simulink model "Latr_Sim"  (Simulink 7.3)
settings: Solver=ode45  StartTime=0.0  StopTime=40  MaxStep=0.01  RelTol=1e-4
InitFcn:
  | % Frequency Response Analysis file Run.m
  | d2r= pi/180; r2d=1/d2r;
  | LQR_des;
  | Mass=8878; Thr=320000;                          % Alpha Estimator parameters
  | Sref= 47.3; Qbar= 220; Cza=-0.31; Cyb=-0.06;
  | [Avf, Bvf, Cvf, Dvf]= vehi_latr_Sflx;          % Load Flex Vehicle Pitch Model
  | load -ascii KMIX.MAT KMIX;                          % Mixing Logic Matrix
  | load -ascii Klat.MAT Klat;                              % LQR Lateral State-Feedback Matrix
StopFcn:
  | Pl
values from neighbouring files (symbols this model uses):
  Aac = [    [actuator.m]
  Bac = [    [actuator.m]
  Cac = [    [actuator.m]
  Dac = [    [actuator.m]
undefined symbols (not defined in the file or in its folder): Avf, Bvf, Cvf, Dvf, Klat, KMIX

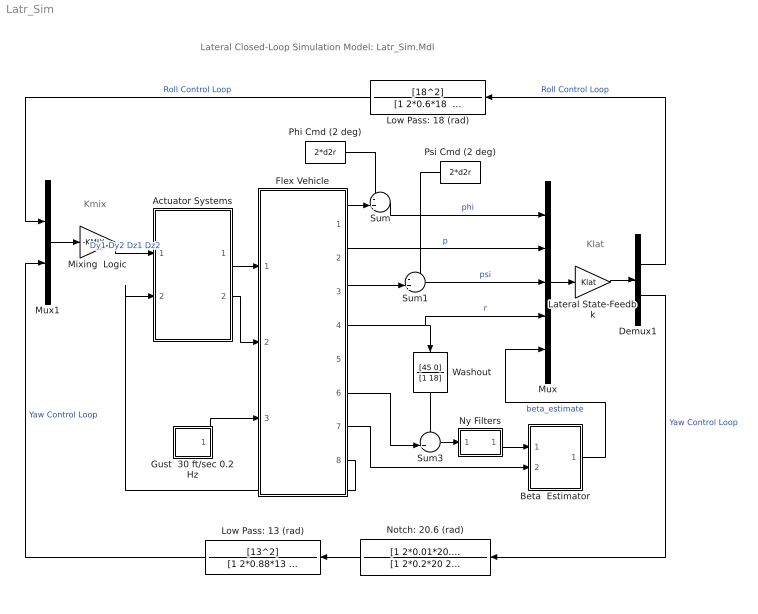
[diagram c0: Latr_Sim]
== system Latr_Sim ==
  note: Lateral Closed-Loop Simulation Model: Latr_Sim.Mdl
  note: Kmix
  note: Klat
  Actuator Systems : Subsystem
  Beta  Estimator : Subsystem
  Demux1 : Demux  Outputs=2
  Flex Vehicle : Subsystem
  Gust  30 ft/sec 0.2 Hz : Subsystem
  Lateral State-Feedbk : Gain  Gain=Klat  Multiplication=Matrix(K*u)  ParameterDataType=sfix(16)  ParameterScaling=2^0  OutDataType=sfix(16)  OutScaling=2^0
  Low Pass: 13 (rad) : TransferFcn  Numerator=[13^2]  Denominator="[1 2*0.88*13  13^2]"
  Low Pass: 18 (rad) : TransferFcn  Numerator=[18^2]  Denominator="[1 2*0.6*18  18^2]"
  Mixing  Logic : Gain  Gain=-KMIX  Multiplication=Matrix(K*u)  ParameterDataType=sfix(16)  ParameterScaling=2^0  OutDataType=sfix(16)  OutScaling=2^0
  Mux : Mux  Inputs=5
  Mux1 : Mux  Inputs=2
  Notch: 20.6 (rad) : TransferFcn  Numerator=[1 2*0.01*20.6 20.6^2]  Denominator=[1 2*0.2*20 20^2]
  Ny Filters : Subsystem
  Phi Cmd (2 deg) : Constant  Value=2*d2r  OutDataType=sfix(16)  OutScaling=2^0
  Psi Cmd (2 deg) : Constant  Value=2*d2r  OutDataType=sfix(16)  OutScaling=2^0
  Sum : Sum  Inputs=-+|  OutDataType=sfix(16)  OutScaling=2^0
  Sum1 : Sum  Inputs=-+|  OutDataType=sfix(16)  OutScaling=2^0
  Sum3 : Sum  Inputs=-+|  OutDataType=sfix(16)  OutScaling=2^0
  Washout : TransferFcn  Numerator=[45 0]  Denominator=[1 18]
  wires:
  Mux/1 -> Lateral State-Feedbk/1
  Lateral State-Feedbk/1 -> Demux1/1
  Mux1/1 -> Mixing  Logic/1
  Flex Vehicle/2(p) -> Mux/2  "p"
  Flex Vehicle/4(r) -> Mux/4, Washout/1  "r"
  Demux1/1 -> Low Pass: 18 (rad)/1  "Roll Control Loop"
  Low Pass: 18 (rad)/1 -> Mux1/1  "Roll Control Loop"
  Low Pass: 13 (rad)/1 -> Mux1/2  "Yaw Control Loop"
  Demux1/2 -> Notch: 20.6 (rad)/1  "Yaw Control Loop"
  Flex Vehicle/1(phi) -> Sum/2
  Sum/1 -> Mux/1  "phi"
  Flex Vehicle/3(psi) -> Sum1/2
  Sum1/1 -> Mux/3  "psi"
  Flex Vehicle/7(DZ) -> Beta  Estimator/2(Dz)
  Sum3/1 -> Ny Filters/1(In)
  Flex Vehicle/6(Ydd) -> Sum3/2
  Gust  30 ft/sec 0.2 Hz/1(Vgust) -> Flex Vehicle/3(Gust)
  Notch: 20.6 (rad)/1 -> Low Pass: 13 (rad)/1
  Ny Filters/1(out) -> Beta  Estimator/1(Ydd)
  Washout/1 -> Sum3/1
  Phi Cmd (2 deg)/1 -> Sum/1
  Psi Cmd (2 deg)/1 -> Sum1/1
  Beta  Estimator/1(bethat) -> Mux/5  "beta_estimate"
  Mixing  Logic/1 -> Actuator Systems/1(deltc)  "Dy1 Dy2 Dz1 Dz2"
  Actuator Systems/1(delta) -> Flex Vehicle/1(deltas)
  Actuator Systems/2(del_dd) -> Flex Vehicle/2(del_ddot)
  Flex Vehicle/8(TL) -> Actuator Systems/2(TL)

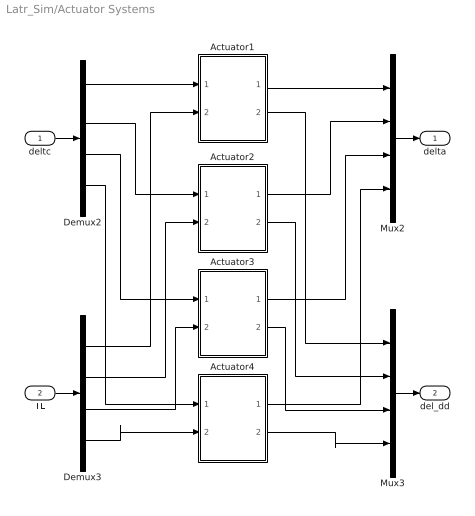
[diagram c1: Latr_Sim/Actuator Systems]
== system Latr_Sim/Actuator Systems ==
  deltc : Inport
  TL : Inport  Port=2
  Actuator1 : Subsystem
  Actuator2 : Subsystem
  Actuator3 : Subsystem
  Actuator4 : Subsystem
  Demux2 : Demux
  Demux3 : Demux
  Mux2 : Mux
  Mux3 : Mux
  delta : Outport
  del_dd : Outport  Port=2
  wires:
  Demux2/1 -> Actuator1/1(Dyc1)
  Demux2/2 -> Actuator2/1(Dyc2)
  Demux2/3 -> Actuator3/1(Dzc1)
  Demux2/4 -> Actuator4/1(Dzc2)
  Demux3/4 -> Actuator4/2(TLz2)
  Demux3/3 -> Actuator3/2(TLz1)
  Demux3/2 -> Actuator2/2(TLy2)
  Demux3/1 -> Actuator1/2(TLy1)
  Actuator1/1(Dy1) -> Mux2/1
  Actuator2/1(Dy2) -> Mux2/2
  Actuator3/1(Dz1) -> Mux2/3
  Actuator4/1(Dz2) -> Mux2/4
  Actuator4/2(Dz_dd2) -> Mux3/4
  Actuator3/2(Dz_dd1) -> Mux3/3
  Actuator2/2(Dy_dd2) -> Mux3/2
  Actuator1/2(Dy_dd1) -> Mux3/1
  deltc/1 -> Demux2/1
  Mux2/1 -> delta/1
  TL/1 -> Demux3/1
  Mux3/1 -> del_dd/1

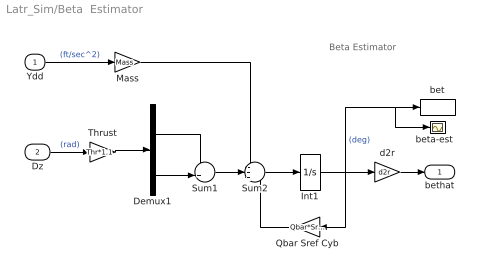
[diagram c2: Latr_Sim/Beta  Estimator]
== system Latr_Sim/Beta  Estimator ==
  note: Beta Estimator
  Ydd : Inport  OutDataType=sfix(16)  OutScaling=2^0
  Dz : Inport  Port=2  OutDataType=sfix(16)  OutScaling=2^0
  Demux1 : Demux  Outputs=2
  Int1 : Integrator
  Mass : Gain  Gain=Mass  ParameterDataType=sfix(16)  ParameterScaling=2^0  OutDataType=sfix(16)  OutScaling=2^0
  Qbar Sref Cyb : Gain  Gain=Qbar*Sref*Cyb  ParameterDataType=sfix(16)  ParameterScaling=2^0  OutDataType=sfix(16)  OutScaling=2^0
  Sum1 : Sum  Inputs=++|  OutDataType=sfix(16)  OutScaling=2^0
  Sum2 : Sum  Inputs=-++  OutDataType=sfix(16)  OutScaling=2^0
  Thrust : Gain  Gain=Thr*1.1  ParameterDataType=sfix(16)  ParameterScaling=2^0  OutDataType=sfix(16)  OutScaling=2^0
  bet : ToWorkspace  VariableName=bethat  SampleTime=-1  SaveFormat=Array
  "beta-est  " : Scope
  d2r : Gain  Gain=d2r  ParameterDataType=sfix(16)  ParameterScaling=2^0  OutDataType=sfix(16)  OutScaling=2^0
  bethat : Outport  OutDataType=sfix(16)  OutScaling=2^0
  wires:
  d2r/1 -> bethat/1
  Mass/1 -> Sum2/1
  Ydd/1 -> Mass/1  "(ft/sec^2)"
  Dz/1 -> Thrust/1  "(rad)"
  Qbar Sref Cyb/1 -> Sum2/3
  Int1/1 -> d2r/1, Qbar Sref Cyb/1, bet/1, "beta-est  "/1  "(deg)"
  Sum1/1 -> Sum2/2
  Sum2/1 -> Int1/1
  Thrust/1 -> Demux1/1
  Demux1/1 -> Sum1/1
  Demux1/2 -> Sum1/2

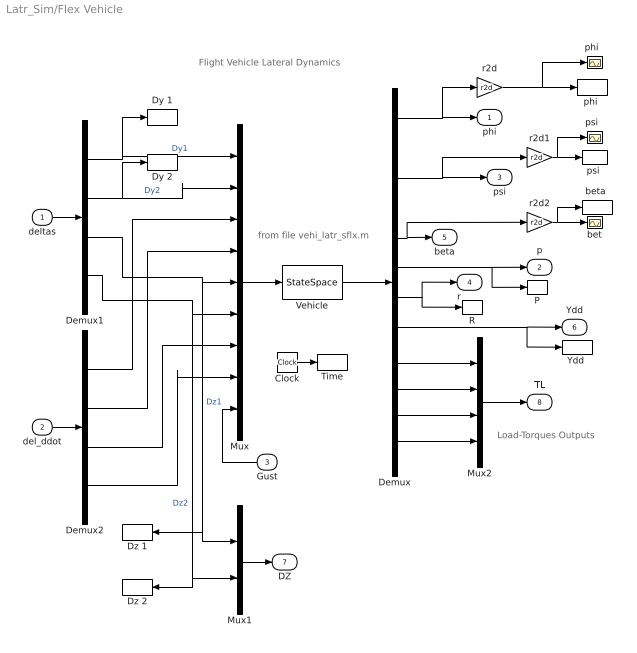
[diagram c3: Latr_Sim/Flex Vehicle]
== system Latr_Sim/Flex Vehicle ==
  note: Flight Vehicle Lateral Dynamics
  note: Load-Torques Outputs
  note: from file vehi_latr_sflx.m
  deltas : Inport  OutDataType=sfix(16)  OutScaling=2^0
  del_ddot : Inport  Port=2  OutDataType=sfix(16)  OutScaling=2^0
  Gust : Inport  Port=3  OutDataType=sfix(16)  OutScaling=2^0
  Clock : Clock
  Demux : Demux  Outputs=12
  Demux1 : Demux
  Demux2 : Demux
  Dy 1 : ToWorkspace  VariableName=Dy1  SampleTime=-1  SaveFormat=Array
  Dy 2 : ToWorkspace  VariableName=Dy2  SampleTime=-1  SaveFormat=Array
  Dz 1 : ToWorkspace  VariableName=Dz1  SampleTime=-1  SaveFormat=Array
  Dz 2 : ToWorkspace  VariableName=Dz2  SampleTime=-1  SaveFormat=Array
  Mux : Mux  Inputs=9
  Mux1 : Mux  Inputs=2
  Mux2 : Mux
  P : ToWorkspace  VariableName=p  SampleTime=-1  SaveFormat=Array
  R : ToWorkspace  VariableName=r  SampleTime=-1  SaveFormat=Array
  Time : ToWorkspace  VariableName=time  SampleTime=-1  SaveFormat=Array
  Vehicle : StateSpace  A=Avf  B=Bvf  C=Cvf  D=Dvf
  "Ydd " : ToWorkspace  VariableName=Ydd  SampleTime=-1  SaveFormat=Array
  bet : Scope
  "beta " : ToWorkspace  VariableName=beta  SampleTime=-1  SaveFormat=Array
  "phi " : ToWorkspace  VariableName=phi  SampleTime=-1  SaveFormat=Array
  "phi  " : Scope
  "psi " : ToWorkspace  VariableName=psi  SampleTime=-1  SaveFormat=Array
  "psi  " : Scope
  r2d : Gain  Gain=r2d  ParameterDataType=sfix(16)  ParameterScaling=2^0  OutDataType=sfix(16)  OutScaling=2^0
  r2d1 : Gain  Gain=r2d  ParameterDataType=sfix(16)  ParameterScaling=2^0  OutDataType=sfix(16)  OutScaling=2^0
  r2d2 : Gain  Gain=r2d  ParameterDataType=sfix(16)  ParameterScaling=2^0  OutDataType=sfix(16)  OutScaling=2^0
  phi : Outport  OutDataType=sfix(16)  OutScaling=2^0
  p : Outport  Port=2  OutDataType=sfix(16)  OutScaling=2^0
  psi : Outport  Port=3  OutDataType=sfix(16)  OutScaling=2^0
  r : Outport  Port=4  OutDataType=sfix(16)  OutScaling=2^0
  beta : Outport  Port=5  OutDataType=sfix(16)  OutScaling=2^0
  Ydd : Outport  Port=6  OutDataType=sfix(16)  OutScaling=2^0
  DZ : Outport  Port=7  OutDataType=sfix(16)  OutScaling=2^0
  TL : Outport  Port=8  OutDataType=sfix(16)  OutScaling=2^0
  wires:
  Mux/1 -> Vehicle/1
  Vehicle/1 -> Demux/1
  deltas/1 -> Demux1/1
  Demux1/1 -> Mux/1, Dy 1/1  "Dy1"
  Demux1/3 -> Mux/5, Mux1/1, Dz 1/1  "Dz1"
  Demux/1 -> phi/1, r2d/1
  Demux/3 -> psi/1, r2d1/1
  Demux/5 -> beta/1, r2d2/1
  Demux/8 -> Ydd/1, "Ydd "/1
  Demux/6 -> p/1, P/1
  Demux1/2 -> Mux/2, Dy 2/1  "Dy2"
  Demux1/4 -> Mux/6, Mux1/2, Dz 2/1  "Dz2"
  Gust/1 -> Mux/9
  r2d/1 -> "phi "/1, "phi  "/1
  r2d1/1 -> "psi "/1, "psi  "/1
  r2d2/1 -> bet/1, "beta "/1
  Demux/7 -> R/1, r/1
  Clock/1 -> Time/1
  Mux1/1 -> DZ/1
  del_ddot/1 -> Demux2/1
  Demux2/1 -> Mux/3
  Demux2/2 -> Mux/4
  Demux2/3 -> Mux/7
  Demux2/4 -> Mux/8
  Demux/9 -> Mux2/1
  Demux/10 -> Mux2/2
  Demux/11 -> Mux2/3
  Demux/12 -> Mux2/4
  Mux2/1 -> TL/1

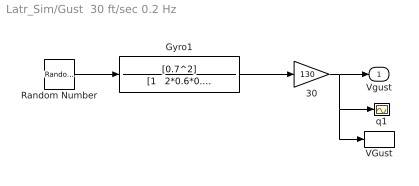
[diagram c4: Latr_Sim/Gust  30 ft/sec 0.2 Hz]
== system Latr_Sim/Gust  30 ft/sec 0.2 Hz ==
  30 : Gain  Gain=130  ParameterDataType=sfix(16)  ParameterScaling=2^0  OutDataType=sfix(16)  OutScaling=2^0
  Gyro1 : TransferFcn  Numerator=[0.7^2]  Denominator="[1   2*0.6*0.7   0.7^2]"
  Random Number : RandomNumber  Seed=-2  SampleTime=0
  VGust : ToWorkspace  VariableName=Vgust  SampleTime=-1  SaveFormat=Array
  q1 : Scope
  Vgust : Outport  OutDataType=sfix(16)  OutScaling=2^0
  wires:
  Gyro1/1 -> 30/1
  30/1 -> Vgust/1, q1/1, VGust/1
  Random Number/1 -> Gyro1/1

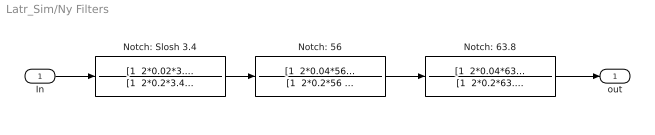
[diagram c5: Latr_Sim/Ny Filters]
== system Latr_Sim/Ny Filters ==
  In : Inport  OutDataType=sfix(16)  OutScaling=2^0
  Notch: 56 : TransferFcn  Numerator="[1  2*0.04*56  56^2]"  Denominator="[1  2*0.2*56  56^2]"
  Notch: 63.8 : TransferFcn  Numerator="[1  2*0.04*63.8  63.8^2]"  Denominator="[1  2*0.2*63.8  63.8^2]"
  Notch: Slosh 3.4 : TransferFcn  Numerator="[1  2*0.02*3.4  3.4^2]"  Denominator="[1  2*0.2*3.4  3.4^2]"
  out : Outport  OutDataType=sfix(16)  OutScaling=2^0
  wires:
  Notch: Slosh 3.4/1 -> Notch: 56/1
  Notch: 56/1 -> Notch: 63.8/1
  Notch: 63.8/1 -> out/1
  In/1 -> Notch: Slosh 3.4/1

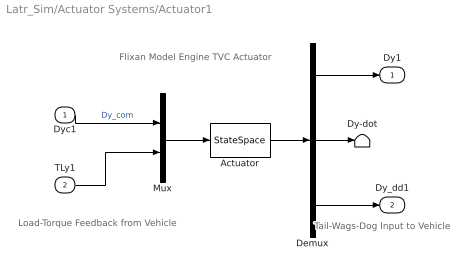
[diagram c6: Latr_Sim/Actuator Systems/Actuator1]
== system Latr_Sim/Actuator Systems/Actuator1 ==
  note: Tail-Wags-Dog Input to Vehicle
  note: Load-Torque Feedback from Vehicle
  note: Flixan Model Engine TVC Actuator
  Dyc1 : Inport  OutDataType=sfix(16)  OutScaling=2^0
  TLy1 : Inport  Port=2  OutDataType=sfix(16)  OutScaling=2^0
  Actuator : StateSpace  A=Aac  B=Bac  C=Cac  D=Dac
  Demux : Demux  Outputs=3
  Dy-dot : Terminator
  Mux : Mux  Inputs=2
  Dy1 : Outport  OutDataType=sfix(16)  OutScaling=2^0
  Dy_dd1 : Outport  Port=2  OutDataType=sfix(16)  OutScaling=2^0
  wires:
  Mux/1 -> Actuator/1
  Actuator/1 -> Demux/1
  Demux/2 -> Dy-dot/1
  Dyc1/1 -> Mux/1  "Dy_com"
  Demux/1 -> Dy1/1
  Demux/3 -> Dy_dd1/1
  TLy1/1 -> Mux/2

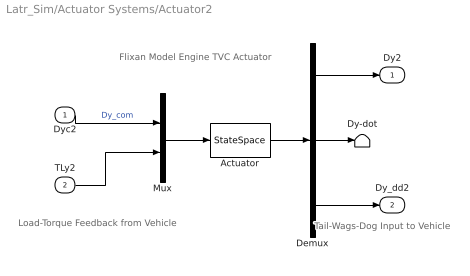
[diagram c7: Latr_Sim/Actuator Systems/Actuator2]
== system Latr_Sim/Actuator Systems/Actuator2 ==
  note: Tail-Wags-Dog Input to Vehicle
  note: Load-Torque Feedback from Vehicle
  note: Flixan Model Engine TVC Actuator
  Dyc2 : Inport  OutDataType=sfix(16)  OutScaling=2^0
  TLy2 : Inport  Port=2  OutDataType=sfix(16)  OutScaling=2^0
  Actuator : StateSpace  A=Aac  B=Bac  C=Cac  D=Dac
  Demux : Demux  Outputs=3
  Dy-dot : Terminator
  Mux : Mux  Inputs=2
  Dy2 : Outport  OutDataType=sfix(16)  OutScaling=2^0
  Dy_dd2 : Outport  Port=2  OutDataType=sfix(16)  OutScaling=2^0
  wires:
  Mux/1 -> Actuator/1
  Actuator/1 -> Demux/1
  Demux/2 -> Dy-dot/1
  Dyc2/1 -> Mux/1  "Dy_com"
  Demux/1 -> Dy2/1
  Demux/3 -> Dy_dd2/1
  TLy2/1 -> Mux/2

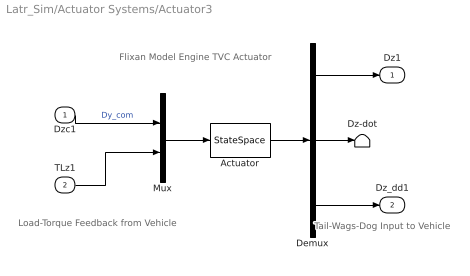
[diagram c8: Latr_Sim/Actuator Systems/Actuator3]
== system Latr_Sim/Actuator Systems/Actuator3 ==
  note: Tail-Wags-Dog Input to Vehicle
  note: Load-Torque Feedback from Vehicle
  note: Flixan Model Engine TVC Actuator
  Dzc1 : Inport  OutDataType=sfix(16)  OutScaling=2^0
  TLz1 : Inport  Port=2  OutDataType=sfix(16)  OutScaling=2^0
  Actuator : StateSpace  A=Aac  B=Bac  C=Cac  D=Dac
  Demux : Demux  Outputs=3
  Dz-dot : Terminator
  Mux : Mux  Inputs=2
  Dz1 : Outport  OutDataType=sfix(16)  OutScaling=2^0
  Dz_dd1 : Outport  Port=2  OutDataType=sfix(16)  OutScaling=2^0
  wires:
  Mux/1 -> Actuator/1
  Actuator/1 -> Demux/1
  Demux/2 -> Dz-dot/1
  Dzc1/1 -> Mux/1  "Dy_com"
  Demux/1 -> Dz1/1
  Demux/3 -> Dz_dd1/1
  TLz1/1 -> Mux/2

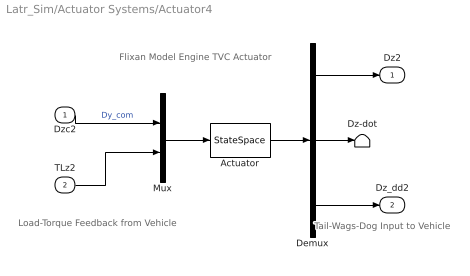
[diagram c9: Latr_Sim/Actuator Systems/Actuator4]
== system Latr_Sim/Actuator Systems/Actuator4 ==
  note: Tail-Wags-Dog Input to Vehicle
  note: Load-Torque Feedback from Vehicle
  note: Flixan Model Engine TVC Actuator
  Dzc2 : Inport  OutDataType=sfix(16)  OutScaling=2^0
  TLz2 : Inport  Port=2  OutDataType=sfix(16)  OutScaling=2^0
  Actuator : StateSpace  A=Aac  B=Bac  C=Cac  D=Dac
  Demux : Demux  Outputs=3
  Dz-dot : Terminator
  Mux : Mux  Inputs=2
  Dz2 : Outport  OutDataType=sfix(16)  OutScaling=2^0
  Dz_dd2 : Outport  Port=2  OutDataType=sfix(16)  OutScaling=2^0
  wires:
  Mux/1 -> Actuator/1
  Actuator/1 -> Demux/1
  Demux/2 -> Dz-dot/1
  Dzc2/1 -> Mux/1  "Dy_com"
  Demux/1 -> Dz2/1
  Demux/3 -> Dz_dd2/1
  TLz2/1 -> Mux/2
